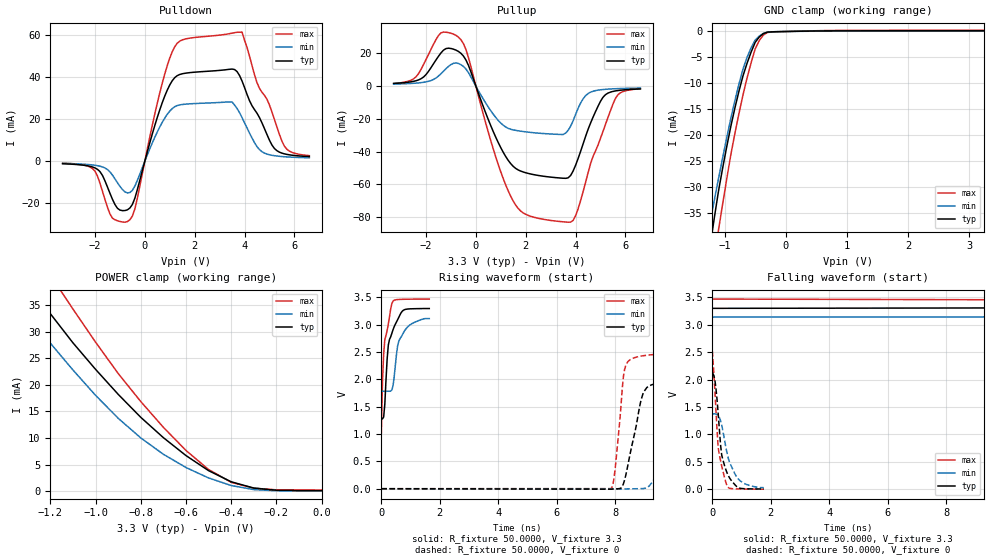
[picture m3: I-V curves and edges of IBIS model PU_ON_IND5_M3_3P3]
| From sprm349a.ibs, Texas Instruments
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|   Model Cell PU_ON_IND5_M3_3P3
|PU_ON_IND5_M3_3P3
[Model]   PU_ON_IND5_M3_3P3
Model_type   I/O
Polarity   Non-Inverting
Enable   Active-Low
Vinl =  0.8V
Vinh =  2V
Cref =  15.0000pF
Rref =  100.0000M
Vref =  0V
Vmeas =  1.65
C_comp   2.519588p   2.450856p   2.584209p
[Model Spec]
Vinl   0.8V   0.8V   0.8V
Vinh   2V   2V   2V
[Temperature Range]   25   125   -40
[Voltage Range]   3.3   3.14   3.47
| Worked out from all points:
|   slope of the pulldown table from 0 to 0.495 V, typ, clamps not added: 24.1 ohm
|   slope of the pullup table from 0 to 0.495 V, typ, clamps not added: 24.3 ohm
|   GND clamp passes 1 mA (typ) near -0.43 V on its own axis
|   POWER clamp passes 1 mA (typ) near -0.33 V on its own axis
|   rising waveform, R_fixture 50.0000, V_fixture 3.3: 20-80 % time 259ps typ, 309ps min, 206ps max; typ from 1.27 V to 3.29 V
|   rising waveform, R_fixture 50.0000, V_fixture 0: 20-80 % time 496ps typ, 2.17ns min, 250ps max; typ from 0 V to 2.12 V
|   falling waveform, R_fixture 50.0000, V_fixture 3.3: 20-80 % time 3.38ns typ, 13.6ns min, 485ps max; typ from 3.3 V to 1.28 V
|   falling waveform, R_fixture 50.0000, V_fixture 0: 20-80 % time 270ps typ, 408ps min, 225ps max; typ from 2.12 V to 0.005 V
[POWER_clamp]
|   voltage   I(typ)   I(min)   I(max)
-3.3V     191.2mA    141.7mA    234.2mA
-1.367V   44.31mA    36.64mA    52.08mA
-1.267V   37.57mA    31.34mA    45.07mA
-1.233V   35.48mA    29.6mA     42.87mA
-1.133V   29.74mA    24.49mA    36.39mA
-1V       22.93mA    18.05mA    28.04mA
-800mV    13.91mA    10.03mA    16.87mA
-600mV    6.717mA    4.468mA    7.675mA
-500mV    3.879mA    2.509mA    4.093mA
-400mV    1.786mA    1.088mA    1.688mA
-300mV    605.1uA    316.8uA    589.7uA
0V        134.4uA    72.62uA    231.1uA
[Pulldown]
|   voltage   I(typ)   I(min)   I(max)
-3.3V     -1.263mA   -1.107mA   -949.2uA
-2.1V     -2.8mA     -1.831mA   -3.557mA
-1.3V     -18.12mA   -6.64mA    -27.06mA
-600mV    -22.25mA   -14.9mA    -27.84mA
-400mV    -17.58mA   -11.86mA   -22.67mA
700mV     27.76mA    18.41mA    37.04mA
1.2V      39.59mA    25.8mA     54.25mA
3.5V      43.66mA    28.02mA    60.67mA
3.9V      37.99mA    20.64mA    61.19mA
4.6V      20.62mA    5.44mA     34.49mA
5.6V      3.432mA    2.063mA    7.065mA
6.6V      2.132mA    1.558mA    2.581mA
[Pullup]
|   voltage   I(typ)   I(min)   I(max)
-3.3V     1.672mA    1.264mA    1.614mA
-2.4V     3.321mA    1.859mA    5.725mA
-1.4V     20.34mA    7.635mA    32.58mA
-700mV    21.21mA    13.85mA    29.95mA
-400mV    16.02mA    10.48mA    22.44mA
1.5V      -49.06mA   -26.73mA   -70.3mA
3.7V      -56.06mA   -27.03mA   -83.17mA
4V        -48.38mA   -17.36mA   -79.25mA
4.4V      -30.79mA   -5.861mA   -58.89mA
5.1V      -6.795mA   -2.058mA   -27.63mA
5.7V      -2.676mA   -1.512mA   -5.259mA
6.6V      -1.699mA   -1.172mA   -1.592mA
[GND_clamp]
|   voltage   I(typ)   I(min)   I(max)
-3.3V     -223.6mA   -167.5mA   -272.3mA
-1.3V     -46.75mA   -40.78mA   -53.98mA
-1.233V   -41.19mA   -36.63mA   -48.64mA
-1.167V   -35.89mA   -32.51mA   -43.44mA
-1.1V     -30.85mA   -28.43mA   -38.37mA
-1.033V   -26.48mA   -24.48mA   -33.43mA
-900mV    -18.42mA   -16.86mA   -23.9mA
-700mV    -8.593mA   -7.272mA   -12.27mA
-500mV    -2.09mA    -1.648mA   -3.35mA
-366.7mV  -404.3uA   -368.4uA   -681.3uA
500mV     94.14uA    54.06uA    144uA
3.233V    134.1uA    76.79uA    229.9uA
[Ramp]
| variable   typ   min   max
dV/dt_f   1.220028/3.362789n   0.8164965/15.5006n   1.484952/0.4554473n
dV/dt_r   1.279632/0.4933797n  0.8206987/1.392243n   1.516757/0.2490544n
R_load = 50
[Rising Waveform]
R_fixture = 50.0000
V_fixture = 3.3
V_fixture_min = 3.14
V_fixture_max = 3.47
|   time   V(typ)   V(min)   V(max)
0s        1.275V     1.779V     1.003V
40ps      1.277V     1.782V     1.96V
80ps      1.31V      1.782V     2.462V
120ps     1.548V     1.782V     2.727V
240ps     2.627V     1.781V     3.014V
360ps     2.839V     1.804V     3.383V
560ps     3.09V      2.619V     3.457V
640ps     3.18V      2.743V     3.46V
1ns       3.287V     3.001V     3.464V
1.64ns    3.292V     3.108V     3.466V
[Rising Waveform]
R_fixture = 50.0000
V_fixture = 0
V_fixture_min = 0
V_fixture_max = 0
|   time   V(typ)   V(min)   V(max)
0s        53.38uV    43.16uV    67.75uV
7.84ns    -8.321mV   108uV      780.1uV
7.96ns    -5.41mV    33.47uV    204.1mV
8.28ns    91.04mV    -5.706mV   2.058V
8.4ns     347.2mV    -3.126mV   2.298V
8.96ns    1.758V     3.192mV    2.43V
10.48ns   2.006V     864.5mV    2.479V
18.72ns   2.083V     1.293V     2.502V
26.68ns   2.091V     1.324V     2.506V
201.8ns   2.12V      1.345V     2.518V
[Falling Waveform]
R_fixture = 50.0000
V_fixture = 3.3
V_fixture_min = 3.14
V_fixture_max = 3.47
|   time   V(typ)   V(min)   V(max)
0s        3.298V     3.138V     3.467V
9.8ns     3.305V     3.142V     3.454V
10ns      3.297V     3.142V     3.036V
10.4ns    2.983V     3.141V     1.587V
10.68ns   2.499V     3.137V     1.407V
11.28ns   1.797V     2.97V      1.32V
13.4ns    1.697V     2.207V     1.187V
19.52ns   1.553V     2.12V      1.079V
75.28ns   1.315V     1.901V     1.006V
263.8ns   1.277V     1.804V     1.003V
[Falling Waveform]
R_fixture = 50.0000
V_fixture = 0
V_fixture_min = 0
V_fixture_max = 0
|   time   V(typ)   V(min)   V(max)
0s        2.124V     1.37V      2.518V
80ps      2.012V     1.375V     1.854V
120ps     1.856V     1.371V     1.459V
200ps     1.373V     1.342V     756.2mV
280ps     813.3mV    1.253V     522.1mV
320ps     621.9mV    1.17V      423.7mV
480ps     329.5mV    716.1mV    92.34mV
600ps     196.8mV    477.4mV    16.25mV
920ps     22.5mV     169.7mV    5.124mV
1.76ns    4.963mV    29.61mV    1.527mV
